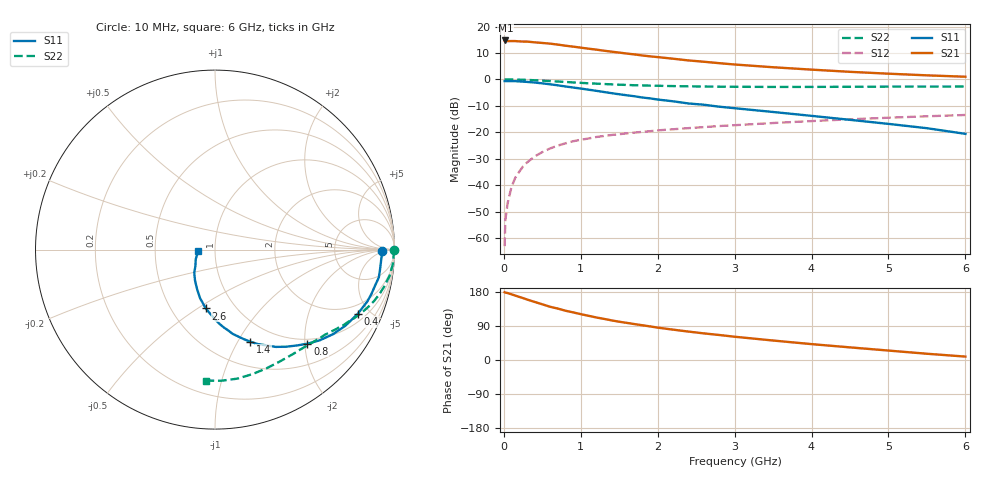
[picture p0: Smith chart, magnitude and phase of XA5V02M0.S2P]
! SIEMENS Discrete & RF Semiconductors
! BFY180
! Si NPN RF Bipolar Junction Transistor in MICRO-X
! VCE = 5 V  IC = 2 mA
! Common Emitter S-Parameters:  May  1997
# GHz  S  MA  R  50
!  f  S11  S21  S12  S22
! GHz  MAG  ANG  MAG  ANG  MAG  ANG  MAG  ANG
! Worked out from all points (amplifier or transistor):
!   36 points, 10 MHz to 6 GHz, reference 50 ohm
!   highest |S21| = 14.7 dB at 20 MHz (marker M1)
!   |S21| within 3 dB of that: start of sweep to 1.071 GHz
!   unconditionally stable (mu >= 1): 2.964 GHz to end of sweep
!   at 250 MHz: K = 0.11, MSG = 23.6 dB, |S12| = -32.9 dB
!   at 1.4 GHz: K = 0.65, MSG = 15.8 dB, |S12| = -21.0 dB
!   at 6 GHz: K = 1.06, MAG = 5.8 dB, |S12| = -13.5 dB
!   S11 on the Smith chart (normalised r, x): 10 MHz: 27, -4; 400 MHz: 1.40, -4.20; 800 MHz: 0.90, -2.06; 1.4 GHz: 0.77, -1.13; 2.6 GHz: 0.73, -0.54; 6 GHz: 0.83, -0.01
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0.01  0.9291 -0.6  5.337 178.8  0.0007 95.5  0.9958 -0.2
0.02  0.9306 -1.2  5.452 178.0  0.0022 91.2  0.9999 -0.6
0.05  0.9281 -3.0  5.302 176.6  0.0046 84.2  0.996 -1.6
0.1  0.9264 -6.3  5.306 173.3  0.0093 87.5  0.9945 -3.3
0.15  0.926 -9.6  5.307 169.9  0.0139 85.3  0.9932 -5.0
0.3  0.8965 -18.8  5.197 159.7  0.0267 78.3  0.9772 -9.7
0.4  0.8719 -24.3  5.023 153.3  0.0348 74.6  0.9636 -12.6
0.6  0.8085 -35.7  4.749 140.5  0.0493 67.9  0.9308 -18.0
0.8  0.735 -45.5  4.34 130.1  0.0616 62.0  0.8937 -22.7
1  0.6713 -53.7  3.987 121.0  0.0721 57.4  0.8601 -26.8
1.1  0.6393 -58.0  3.81 116.7  0.0762 55.6  0.8441 -28.5
1.4  0.5489 -69.1  3.345 104.6  0.0888 51.0  0.8059 -33.5
1.6  0.5008 -75.1  3.079 97.9  0.0953 48.7  0.7852 -36.3
1.8  0.4541 -81.0  2.836 91.7  0.1018 46.8  0.7689 -39.1
2  0.4161 -86.3  2.642 85.4  0.1086 44.6  0.7572 -41.7
2.2  0.385 -90.5  2.461 80.1  0.1139 42.9  0.7469 -44.4
2.6  0.3317 -99.0  2.158 70.2  0.1251 39.9  0.7323 -49.4
3  0.285 -106.8  1.913 61.4  0.136 37.1  0.7247 -54.3
3.5  0.2418 -114.4  1.697 51.4  0.1495 33.8  0.7203 -60.4
4.5  0.1718 -132.3  1.39 33.3  0.1759 26.7  0.7244 -73.3
5.5  0.1193 -153.9  1.193 16.5  0.2006 19.2  0.7315 -87.1
6  0.0933 -175.2  1.123 9.0  0.2122 14.9  0.7318 -94.1
